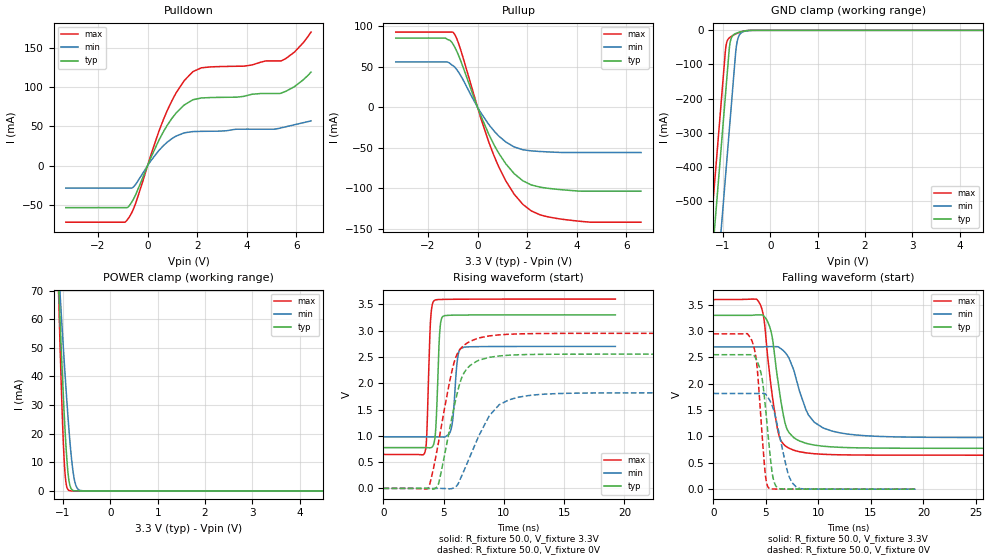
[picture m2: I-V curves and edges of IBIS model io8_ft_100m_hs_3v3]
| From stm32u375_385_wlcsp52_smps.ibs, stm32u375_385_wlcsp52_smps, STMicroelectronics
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[Model]   io8_ft_100m_hs_3v3
Model_type I/O
Polarity   Non-Inverting
Enable   Active-Low
| CAP_THRESHOLD on pad IOFT is "UDTCAPC" :
| Rising=30.0% of vddiom   Falling=70.0% of vddiom
| C_comp min and max val. don't necessarily correlate with the min and max pvt
| but are the smallest and greatest pad capacitance found.
| var   typ   min   max
C_comp   3.79549pF  3.74406pF  3.79817pF
|C_comp_pullup   2.32818pF  2.17341pF  2.40238pF
|C_comp_pulldown   1.46732pF  1.57065pF  1.39579pF
Vinl = 1.35V
Vinh = 1.8V
Vmeas = 1.65V   | Reference voltage for timing measurements
Cref  = 50.0pF   | Timing specification test load capacitance value
Rref  = 1.0MOhm   | Timing specification test load resistance value
Vref  = 1.815V   | Timing specification test load voltage
[Model Spec]
| TIME_THRESHOLD on pin ZIV11 is "CMOS" :
| Rising=50.0% of vdd   Falling=50.0% of vdd
Vinl 1.27950V 1.06950V 1.36550V
Vinh 1.78950V 1.51350V 1.89450V
| variable   typ   min   max
[Temperature Range] 25.0 130.0 -40.0
| variable   typ   min   max
[Voltage Range] 3.3V 2.7V 3.6V
| variable   typ   min   max
[POWER Clamp Reference] 3.3V 2.7V 3.6V
| variable   typ   min   max
[GND Clamp Reference] 0V 0V 0V
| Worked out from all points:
|   slope of the pulldown table from 0 to 0.495 V, typ, clamps not added: 14.3 ohm
|   slope of the pullup table from 0 to 0.495 V, typ, clamps not added: 13.8 ohm
|   GND clamp passes 1 mA (typ) near -0.50 V on its own axis
|   POWER clamp passes 1 mA (typ) near -0.83 V on its own axis
|   rising waveform, R_fixture 50.0, V_fixture 3.3V: 20-80 % time 252ps typ, 335ps min, 240ps max; typ from 0.776 V to 3.3 V
|   falling waveform, R_fixture 50.0, V_fixture 3.3V: 20-80 % time 1.13ns typ, 1.92ns min, 1.08ns max; typ from 3.3 V to 0.776 V
|   rising waveform, R_fixture 50.0, V_fixture 0V: 20-80 % time 1.44ns typ, 2.34ns min, 1.49ns max; typ from 0 V to 2.55 V
|   falling waveform, R_fixture 50.0, V_fixture 0V: 20-80 % time 791ps typ, 1.22ns min, 669ps max; typ from 2.55 V to 0 V
[POWER Clamp]
-3.3V     1.126A     769.5mA    1.647A
-1.1V     75.38mA    79.63mA    73.18mA
-1.09V    71.2mA     76.8mA     67.14mA
-1.08V    67.05mA    73.98mA    61.2mA
-1.06V    58.89mA    68.38mA    49.67mA
-1.01V    39.47mA    54.71mA    24.03mA
-970mV    25.49mA    44.18mA    9.257mA
-930mV    13.81mA    34.16mA    2.168mA
-870mV    3.251mA    20.56mA    140.6uA
-760mV    67.19uA    3.98mA     739.8nA
-630mV    518.7nA    149.1uA    1.803nA
6.6V      0A         0A         0A
[GND Clamp]
-3.3V     -4.191A    -4.432A    -4.059A
-1.25V    -706mA     -946.8mA   -573.6mA
-950mV    -196mA     -436.8mA   -63.63mA
-940mV    -179mA     -419.8mA   -50.26mA
-910mV    -128mA     -368.8mA   -31.05mA
-850mV    -37.37mA   -266.8mA   -20.53mA
-810mV    -18.79mA   -198.8mA   -16.88mA
-720mV    -8.735mA   -51.28mA   -10.12mA
-680mV    -6.635mA   -22.61mA   -7.598mA
-630mV    -4.51mA    -9.474mA   -4.925mA
-400mV    -114.4uA   -369.6uA   -46.93uA
6.6V      2.22nA     299.7nA    1.002nA
| variable   typ   min   max
[Pullup Reference] 3.3V 2.7V 3.6V
| variable   typ   min   max
[Pulldown Reference] 0V 0V 0V
[Pullup]
-3.3V     85.47mA    55.95mA    92.79mA
-1.31V    85.47mA    55.95mA    92.79mA
-950mV    75.9mA     50.36mA    91.24mA
-710mV    59.85mA    40.58mA    73.66mA
120mV     -9.578mA   -6.208mA   -12.33mA
650mV     -45.52mA   -28.81mA   -58.82mA
1.14V     -69.93mA   -42.96mA   -90.97mA
1.83V     -90.96mA   -52.61mA   -120.1mA
2.51V     -98.71mA   -54.73mA   -132.8mA
3.3V      -101.8mA   -55.87mA   -138mA
4.55V     -103.8mA   -56.04mA   -142.1mA
6.6V      -103.8mA   -56.04mA   -142.1mA
[Pulldown]
-3.3V     -53.27mA   -28.52mA   -71.84mA
-840mV    -53.27mA   -28.52mA   -69.65mA
-500mV    -38.18mA   -24.47mA   -49.51mA
460mV     32.61mA    19.53mA    43.99mA
800mV     51.7mA     30.09mA    70.55mA
1.14V     66.56mA    37.47mA    92mA
1.48V     77.24mA    41.82mA    108.3mA
1.83V     83.91mA    43.43mA    119.6mA
2.17V     86.16mA    43.73mA    124.5mA
5.39V     92.36mA    48.12mA    133.3mA
5.93V     100.6mA    52.1mA     144.5mA
6.6V      119.1mA    57.05mA    170mA
[Ramp]
dV/dt_r 1.53141V/1.43453ns 1.09015V/2.27316ns 1.76896V/1.48949ns
dV/dt_f 1.51461V/1.12409ns 1.03188V/1.84199ns 1.77292V/1.08052ns
R_load = 50.0
| Removed startup time: 0s 0s 0s  .
| Removed end time: 19.25ns.
[Rising Waveform]
R_fixture   = 50.0
V_fixture   = 3.3V
V_fixture_min = 2.7V
V_fixture_max = 3.6V
0s        775.7mV    980.2mV    645.1mV
3.45ns    775.7mV    980.2mV    694.1mV
3.6ns     775.5mV    980.2mV    1.054V
3.9ns     772.2mV    980.2mV    3.175V
4.25ns    925mV      980.2mV    3.577V
4.65ns    2.913V     979.9mV    3.591V
4.95ns    3.273V     977mV      3.594V
5.65ns    3.293V     1.16V      3.596V
6.4ns     3.296V     2.659V     3.597V
19.25ns   3.3V       2.7V       3.6V
| Removed startup time: 0s 0s 0s  .
| Removed end time: 39.25ns.
[Falling Waveform]
R_fixture   = 50.0
V_fixture   = 3.3V
V_fixture_min = 2.7V
V_fixture_max = 3.6V
0s        3.3V       2.7V       3.6V
4.45ns    3.308V     2.7V       3.509V
4.85ns    3.276V     2.703V     3.171V
5.45ns    3.018V     2.706V     2.013V
6.15ns    2.045V     2.702V     1.094V
6.85ns    1.234V     2.589V     822.1mV
7.65ns    978mV      2.262V     739.5mV
9.05ns    858.9mV    1.407V     683.4mV
12.05ns   794.2mV    1.069V     652.3mV
39.25ns   775.7mV    980.2mV    645.1mV
| Removed startup time: 0s 0s 0s  .
| Removed end time: 39.2ns.
[Rising Waveform]
R_fixture   = 50.0
V_fixture   = 0V
V_fixture_min = 0V
V_fixture_max = 0V
0s        11.22nV    82.64nV    22.9nV
3.75ns    -1.955mV   2.959uV    20.28mV
4.55ns    73.95mV    90.57uV    856.4mV
5.45ns    1.081V     -8.278mV   1.983V
5.95ns    1.64V      23.61mV    2.46V
6.65ns    2.181V     321.3mV    2.715V
7.75ns    2.419V     912.3mV    2.848V
9.6ns     2.518V     1.589V     2.919V
12ns      2.546V     1.764V     2.942V
39.2ns    2.552V     1.817V     2.948V
| Removed startup time: 0s 0s 0s  .
| Removed end time: 19.25ns.
[Falling Waveform]
R_fixture   = 50.0
V_fixture   = 0V
V_fixture_min = 0V
V_fixture_max = 0V
0s        2.552V     1.817V     2.948V
3.7ns     2.555V     1.817V     2.797V
4.15ns    2.436V     1.817V     2.33V
4.6ns     2.135V     1.817V     1.119V
4.95ns    1.558V     1.805V     264.5mV
5.3ns     832.8mV    1.707V     15.83mV
5.95ns    60.13mV    1.333V     2.627mV
7.1ns     2.373mV    301.9mV    1.36mV
7.9ns     1.56mV     38.81mV    1.042mV
19.25ns   29.23uV    82.76uV    25.98uV
